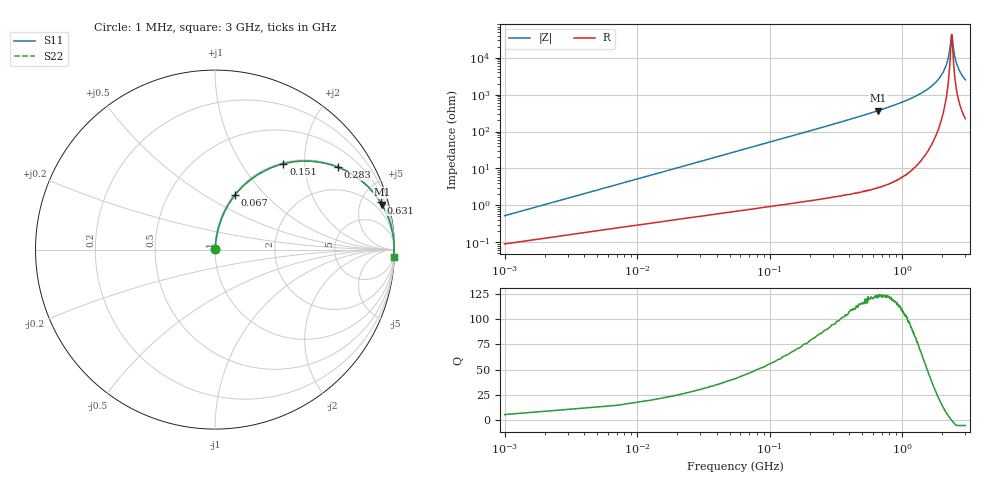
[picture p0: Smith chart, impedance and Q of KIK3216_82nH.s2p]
!version-2
!date-01.2022
!Series
# MHz S RI R 50
!Freq ReS11 ImS11 ReS21 ImS21 ReS12 ImS12 ReS22 ImS22
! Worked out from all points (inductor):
!   501 points, 1 MHz to 3 GHz, reference 50 ohm
!   read as one part in series: L = 82 nH near 13 MHz
!   highest Q = 123 at 661 MHz (marker M1), where L = 89 nH
!   self-resonance near 2.36 GHz
!   S11 on the Smith chart (normalised r, x): 1 MHz: 1.00, +0.01; 67 MHz: 1.02, +0.69; 151 MHz: 1.02, +1.56; 283 MHz: 1.03, +2.96; 631 MHz: 1.06, +7.00; 3 GHz: 5, -50
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1  0.000948 0.00514  0.9991 -0.00514  0.9991 -0.00514  0.000948 0.00514
19  0.0134 0.0962  0.9866 -0.0962  0.9866 -0.0962  0.0134 0.0962
25  0.0207 0.1256  0.9793 -0.1256  0.9793 -0.1256  0.0207 0.1256
43  0.052 0.2088  0.948 -0.2088  0.948 -0.2088  0.052 0.2088
67  0.1119 0.3045  0.8881 -0.3045  0.8881 -0.3045  0.1119 0.3045
151  0.3807 0.4783  0.6193 -0.4783  0.6193 -0.4783  0.3807 0.4783
283  0.6845 0.4593  0.3155 -0.4593  0.3155 -0.4593  0.6845 0.4593
505  0.8793 0.3215  0.1207 -0.3215  0.1207 -0.3215  0.8793 0.3215
631  0.9227 0.263  0.0773 -0.263  0.0773 -0.263  0.9227 0.263
661  0.93 0.2511  0.07 -0.2511  0.07 -0.2511  0.93 0.2511
1010  0.9745 0.153  0.0255 -0.153  0.0255 -0.153  0.9745 0.153
1505  0.9927 0.0765  0.0073 -0.0765  0.0073 -0.0765  0.9927 0.0765
1800  0.9963 0.0455  0.0037 -0.0455  0.0037 -0.0455  0.9963 0.0455
2005  0.9974 0.027  0.00258 -0.027  0.00258 -0.027  0.9974 0.027
2220  0.9978 0.0106  0.00222 -0.0106  0.00222 -0.0106  0.9978 0.0106
2280  0.9978 0.00624  0.00224 -0.00624  0.00224 -0.00624  0.9978 0.00624
2360  0.9977 0.000309  0.00232 -0.000309  0.00232 -0.000309  0.9977 0.000309
2380  0.9977 -0.000933  0.00235 0.000933  0.00235 0.000933  0.9977 -0.000933
2430  0.9975 -0.0046  0.00245 0.0046  0.00245 0.0046  0.9975 -0.0046
2505  0.9974 -0.00937  0.00264 0.00937  0.00264 0.00937  0.9974 -0.00937
2670  0.9968 -0.02  0.00324 0.02  0.00324 0.02  0.9968 -0.02
3000  0.995 -0.0392  0.00501 0.0392  0.00501 0.0392  0.995 -0.0392
